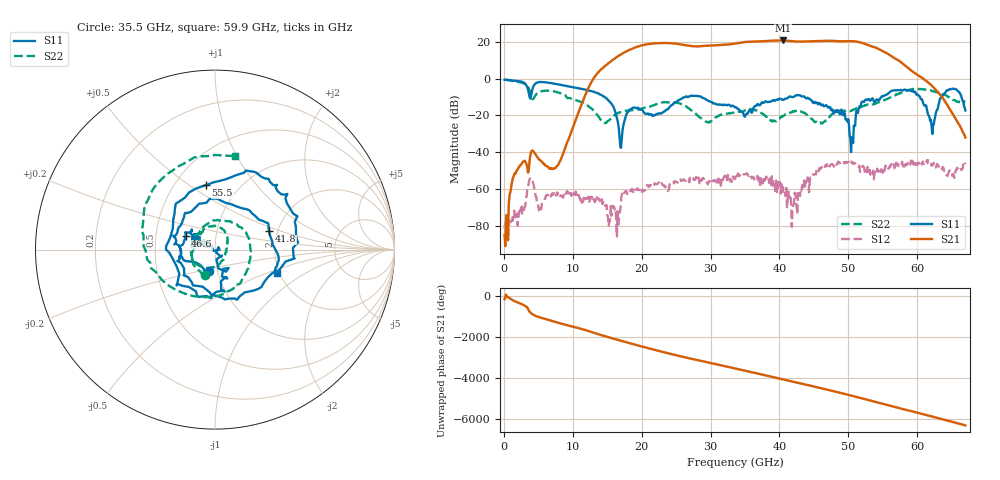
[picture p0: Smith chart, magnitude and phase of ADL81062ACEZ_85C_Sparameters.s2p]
! Analog Devices Inc.
! Device:  ADL81062ACEZ
! Description: GaAs pHEMT Low Noise Amplifier.
! Frequency:  18.00 -  54.00 GHz
! Package:
! Conditions:	Vdd = 3.0 V
!		Idd = 120 mA
!		Temp = +85 C
! Calibration: Board loss de-embedded from S21 magnitude. All other RF measurements reference to RF coaxial connector
! Misc:DB
! Freq(GHz)	S11a(dB)	S11p(deg)	S21a(dB)	S21p(deg)	S12a(dB)	S12p(deg)	S22a(dB)	S22p(deg)
# GHz S  dB  R 50
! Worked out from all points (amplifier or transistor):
!   670 points, 100 MHz to 67 GHz, reference 50 ohm
!   highest |S21| = 20.8 dB at 40.5 GHz (marker M1)
!   |S21| within 3 dB of that: 29.03 GHz to 53.25 GHz (24.21 GHz wide, 58.9 % of centre)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
!   unconditionally stable (mu >= 1): start of sweep to end of sweep
!   at 11.2 GHz: K = 3077.18, MAG = -13.0 dB, |S12| = -64.5 dB
!   at 33.6 GHz: K = 27.27, MAG = 19.4 dB, |S12| = -54.3 dB
!   at 67 GHz: K = 3544.29, MAG = -31.7 dB, |S12| = -45.7 dB
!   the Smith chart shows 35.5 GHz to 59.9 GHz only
!   S11 on the Smith chart (normalised r, x): 35.5 GHz: 0.91, -0.22; 41.8 GHz: 1.80, +0.41; 46.6 GHz: 0.71, +0.11; 55.5 GHz: 0.70, +0.58; 59.9 GHz: 1.95, -0.58
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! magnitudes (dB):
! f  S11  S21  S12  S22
! 100 MHz  -0.5  -85.0  -81.9  -0.6
! 1.5 GHz  -1.0  -52.1  -71.7  -1.5
! 3.9 GHz  -10.0  -40.5  -53.9  -8.8
! 5.1 GHz  -1.8  -43.9  -71.6  -7.2
! 7.6 GHz  -2.9  -47.9  -63.6  -7.2
! 11.3 GHz  -5.5  -13.7  -67.5  -12.9
! 17 GHz  -37.6  13.3  -66.8  -18.2
! 22.4 GHz  -19.0  19.4  -56.9  -13.6
! 33.6 GHz  -15.6  19.2  -54.3  -17.9
! 35.5 GHz  -18.0  20.1  -52.5  -16.3
! 40.5 GHz  -11.4  20.8  -58.9  -20.3
! 41.8 GHz  -9.9  20.5  -80.7  -18.1
! 44.7 GHz  -11.9  20.4  -53.1  -21.8
! 46.6 GHz  -14.9  20.6  -47.8  -23.1
! 50.5 GHz  -31.9  20.5  -45.8  -17.5
! 51.9 GHz  -13.0  19.6  -49.1  -15.3
! 55.5 GHz  -8.8  14.1  -48.3  -11.2
! 55.9 GHz  -7.7  13.2  -48.9  -10.5
! 59.9 GHz  -8.6  2.5  -46.0  -5.5
! 62.2 GHz  -30.1  -4.0  -46.5  -6.8
! 64.5 GHz  -6.3  -15.1  -51.8  -9.9
! 67 GHz  -17.3  -32.0  -45.7  -12.3
